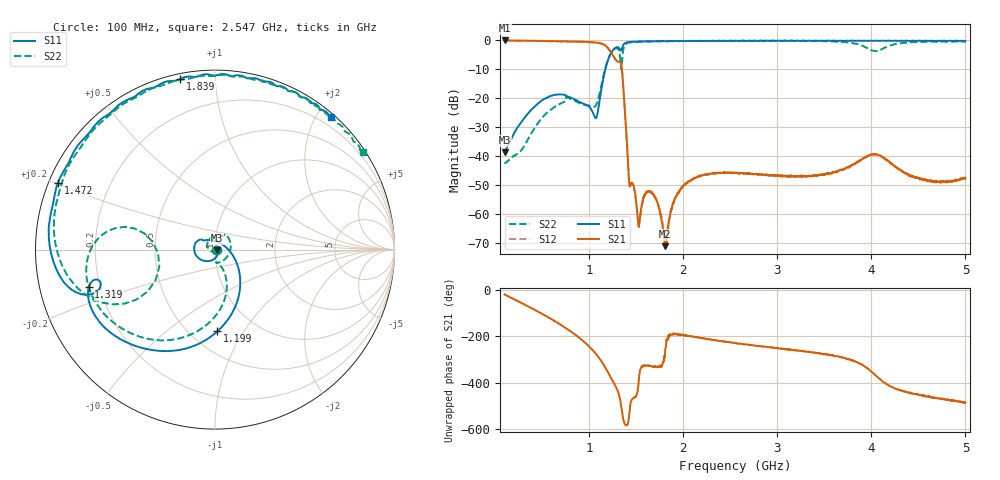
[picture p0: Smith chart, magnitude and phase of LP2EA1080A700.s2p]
!Agilent Technologies,E8358A,US41080443,A.07.50.56
!Agilent E8358A: A.07.50.56
!Date: Monday, April 17, 2017 09:23:51
!Correction: S11(Full 2 Port(1,2))
!S21(Full 2 Port(1,2))
!S12(Full 2 Port(1,2))
!S22(Full 2 Port(1,2))
!S2P File: Measurements: S11, S21, S12, S22:
# Hz S  dB  R 50
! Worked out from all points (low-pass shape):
!   1601 points, 100 MHz to 5 GHz, reference 50 ohm
!   highest |S21| = -0.02 dB at 100 MHz (marker M1); lowest = -71.1 dB at 1.803 GHz (marker M2)
!   |S21| within 3 dB of the highest: start of sweep to 1.209 GHz
!   lowest |S11| = -38.7 dB at 100 MHz (marker M3), VSWR 1.02, Z = 51.1 - j0.346 ohm
!   |S11| at or under -10 dB: start of sweep to 1.171 GHz
!   |S22| runs from -42.6 to -0.1 dB; largest |S21 - S12| = 0.011
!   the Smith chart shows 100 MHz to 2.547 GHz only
!   S11 on the Smith chart (normalised r, x): 100 MHz: 1.02, -0.01; 1.199 GHz: 0.67, -0.77; 1.319 GHz: 0.16, -0.14; 1.472 GHz: 0.03, +0.20; 1.839 GHz: 0.02, +0.82; 2.547 GHz: 0.06, +2.21
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1e8  -38.71 -17.0  -0.02 -20.2  -0.11 -20.1  -42.59 -9.6
5.073125e8  -20.54 -141.3  -0.19 -105.3  -0.27 -105.2  -26.42 153.4
7.43125e8  -18.86 160.2  -0.35 -162.5  -0.43 -162.4  -21.09 62.3
9.176875e8  -21.61 141.7  -0.46 145.6  -0.54 145.7  -22.06 -29.1
1.076938e9  -26.67 49.3  -0.74 81.3  -0.84 81.5  -22.04 -77.5
1.199438e9  -6.83 -88.3  -2.65 4.4  -2.74 4.6  -6.69 -101.9
1.318875e9  -2.69 -163.4  -7.39 -95.1  -7.48 -94.8  -3.94 172.7
1.426062e9  -0.57 169.0  -49.64 -172.6  -49.62 -172.9  -0.75 166.0
1.472e9  -0.43 156.9  -50.24 -105.2  -50.50 -106.2  -0.54 151.1
1.530188e9  -0.37 144.5  -63.55 -19.8  -64.29 -18.4  -0.45 136.8
1.735375e9  -0.25 112.8  -56.96 27.1  -56.97 28.9  -0.30 101.4
1.80275e9  -0.24 104.9  -71.13 68.9  -68.31 91.6  -0.27 92.8
1.8395e9  -0.25 101.4  -64.91 162.2  -64.06 161.0  -0.26 88.9
2.032438e9  -0.21 83.4  -49.40 163.4  -49.65 163.8  -0.20 69.6
2.546938e9  -0.16 48.8  -45.72 131.4  -45.94 132.1  -0.12 33.5
2.55e9  -0.15 48.5  -45.73 131.0  -45.99 131.3  -0.10 33.2
3.367688e9  -0.18 13.2  -46.88 90.2  -47.06 90.5  -0.25 -10.3
3.8975e9  -0.17 -2.5  -41.14 38.4  -41.09 37.9  -1.75 -90.1
4.035312e9  -0.14 -6.1  -39.33 -4.5  -39.38 -4.4  -3.65 177.9
4.185375e9  -0.08 -10.6  -41.81 -51.8  -41.97 -51.5  -1.92 75.6
4.451812e9  -0.11 -17.7  -47.25 -87.7  -47.15 -89.1  -0.56 14.4
5e9  -0.20 -32.0  -47.78 -126.5  -47.61 -125.0  -0.47 -37.3
